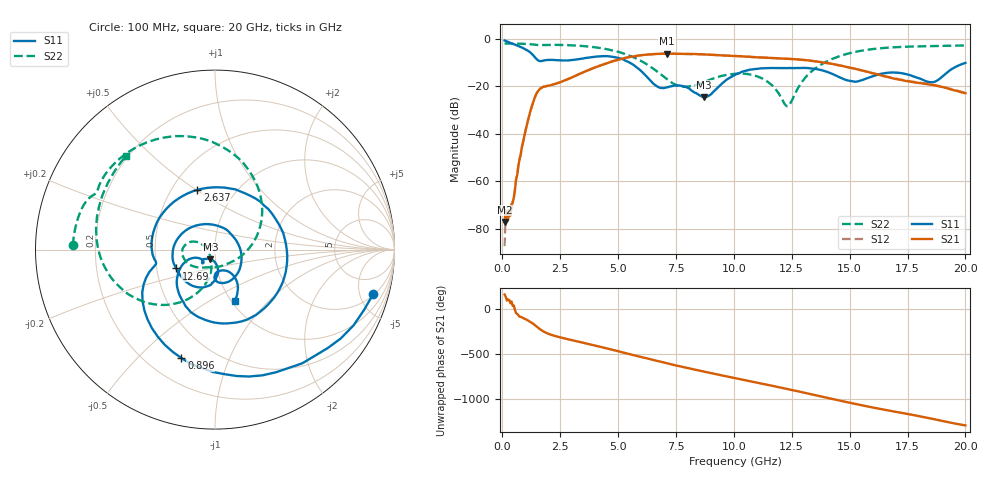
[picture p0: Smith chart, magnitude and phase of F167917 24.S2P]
!  2-Port S-parameters saved by WinCal
! VAR MeasName=S-Parameters (CALIBRATED_DATA) read from VNA (N5242A)
! VAR MeasDate=2016-11-22 9:00:53
! VAR NAME=F167917 24
! VAR FILENAME=F167917 24.S2P
! VAR DATE=2016-11-22 9:00:53
! VAR PHYS_PORTS=1,2
# Hz S DB R 50
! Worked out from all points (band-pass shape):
!   401 points, 100 MHz to 20 GHz, reference 50 ohm
!   highest |S21| = -6.32 dB at 7.115 GHz (marker M1); lowest = -77.2 dB at 100 MHz (marker M2)
!   |S21| within 3 dB of the highest: 4.84 GHz to 13.34 GHz (8.496 GHz wide, 93.5 % of centre)
!   lowest |S11| = -24.6 dB at 8.707 GHz (marker M3), VSWR 1.13, Z = 47.2 - j5.05 ohm
!   |S11| at or under -10 dB: 5.485 GHz to end of sweep
!   |S22| runs from -28.5 to -2.0 dB; largest |S21 - S12| = 0.0047
!   S11 on the Smith chart (normalised r, x): 100 MHz: 2.17, -6.64; 896 MHz: 0.34, -0.68; 2.637 GHz: 0.67, +0.51; 12.69 GHz: 0.63, -0.14; 20 GHz: 1.03, -0.66
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1e8  -0.76 -15.5  -77.16 162.0  -87.35 -160.3  -2.02 178.3
4.4825e8  -2.19 -57.8  -69.06 36.4  -67.85 47.0  -2.06 172.4
8.96e8  -3.98 -107.2  -43.59 -97.8  -43.57 -97.3  -2.16 164.7
1.54275e9  -9.11 -164.8  -22.09 155.0  -22.02 155.0  -2.69 154.7
2.63725e9  -9.18 106.3  -17.83 39.2  -17.80 38.9  -2.67 137.1
3.43325e9  -8.46 27.4  -14.44 -8.3  -14.44 -8.4  -3.08 120.1
3.9805e9  -7.62 -21.8  -12.22 -41.4  -12.21 -41.4  -3.61 106.6
4.677e9  -7.53 -76.7  -9.77 -84.8  -9.73 -84.8  -4.77 86.8
5.5725e9  -10.48 -134.5  -7.62 -142.9  -7.59 -143.0  -7.43 56.1
6.7665e9  -20.51 -147.0  -6.39 141.4  -6.39 141.2  -14.43 2.1
7.11475e9  -20.47 -133.0  -6.32 120.1  -6.33 120.1  -17.06 -18.8
7.861e9  -20.12 -136.6  -6.43 76.5  -6.41 76.6  -20.25 -77.8
8.70675e9  -24.58 -115.6  -6.62 28.9  -6.62 28.8  -18.31 -124.4
1.005e10  -15.26 -91.0  -7.30 -43.4  -7.29 -43.2  -14.86 -166.2
1.13435e10  -12.42 -124.9  -8.02 -111.9  -7.96 -111.7  -17.36 160.9
1.228875e10  -12.40 -145.2  -8.46 -162.6  -8.41 -162.8  -28.45 -159.9
1.268675e10  -12.38 -154.0  -8.69 175.6  -8.68 175.2  -22.32 -104.2
1.338325e10  -12.55 -177.4  -9.34 135.5  -9.35 135.3  -13.56 -106.7
1.51245e10  -17.94 54.3  -12.41 37.9  -12.45 38.2  -5.83 -147.1
1.67165e10  -14.30 -62.6  -16.28 -43.6  -16.25 -42.7  -3.75 -179.9
1.8607e10  -18.30 -72.5  -19.56 -135.9  -19.43 -135.6  -3.11 151.2
2e10  -10.20 -69.3  -22.98 152.6  -22.78 152.9  -2.88 133.5
